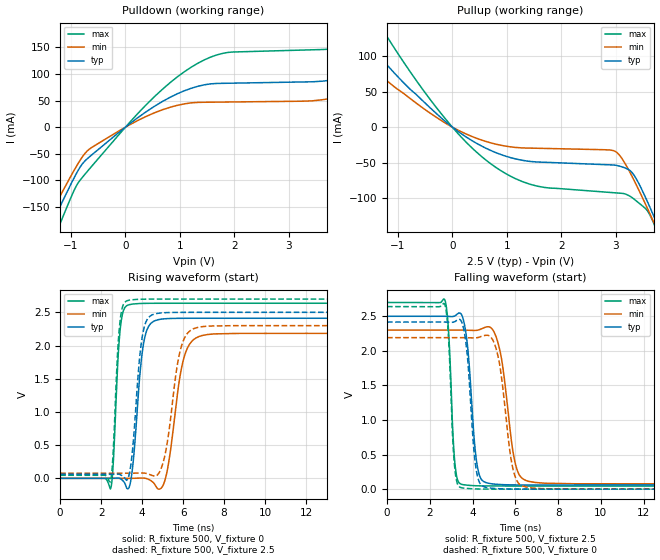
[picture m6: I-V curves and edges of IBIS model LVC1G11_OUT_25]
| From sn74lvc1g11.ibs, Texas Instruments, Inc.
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[Model]   LVC1G11_OUT_25
Model_type  Output
Vref =   0
Rref =   500
Cref =   30p
Vmeas =   1.25
| variable   typ   min   max
C_comp   8.68pF   6.47pF   11.64pF
| C_pullup   8.47pF   6.47pF   9.44pF
| C_pulldown   8.88pF   6.52pF   11.64pF
[Temperature Range]   40   100   -40
| Ambient temperature   25   85   -40
[Voltage range]   2.5   2.3   2.7
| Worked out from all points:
|   slope of the pulldown table from 0 to 0.375 V, typ, clamps not added: 13.1 ohm
|   slope of the pullup table from 0 to 0.375 V, typ, clamps not added: 19.1 ohm
|   rising waveform, R_fixture 500, V_fixture 0: 20-80 % time 389ps typ, 592ps min, 250ps max; typ from 0 V to 2.41 V
|   falling waveform, R_fixture 500, V_fixture 2.5: 20-80 % time 346ps typ, 532ps min, 224ps max; typ from 2.5 V to 0.06 V
|   rising waveform, R_fixture 500, V_fixture 2.5: 20-80 % time 383ps typ, 591ps min, 246ps max; typ from 0.06 V to 2.5 V
|   falling waveform, R_fixture 500, V_fixture 0: 20-80 % time 334ps typ, 507ps min, 221ps max; typ from 2.42 V to 0 V
[Pulldown]
| LVC1G11_OUT_25
|   Voltage   I(typ)   I(min)   I(max)
-5.5V     -1.065A    -962.2mA   -1.233A
-1.515V   -217.8mA   -190.9mA   -261.5mA
-1.145V   -137.3mA   -118.9mA   -167.6mA
-660mV    -55.79mA   -41.12mA   -78.48mA
535mV     39.4mA     27.09mA    57.66mA
1.455V    79.8mA     46.83mA    127mA
3.83V     89.86mA    55.41mA    148.1mA
5.34V     157.5mA    105.9mA    231.7mA
5.91V     188.7mA    52.63mA    283.1mA
6.525V    93.57mA    53.14mA    299.2mA
7.56V     94.12mA    54.12mA    161mA
11V       99.65mA    57.57mA    169.2mA
[Pullup]
| LVC1G11_OUT_25
|   Voltage   I(typ)   I(min)   I(max)
-5.5V     548.1mA    433.4mA    764.5mA
-2.31V    190.8mA    146mA      272.9mA
-1.86V    147mA      111.5mA    211.6mA
-1.295V   95.71mA    71.6mA     139.1mA
-180mV    11.41mA    8.219mA    16.71mA
710mV     -33.04mA   -22.25mA   -51.89mA
1.555V    -49.16mA   -29.78mA   -83.08mA
2.995V    -53.63mA   -34.3mA    -92.61mA
3.34V     -67.98mA   -75.27mA   -101.5mA
3.565V    -101.9mA   -111.4mA   -116.1mA
3.76V     -136.1mA   -144.4mA   -146.6mA
11V       -1.614A    -1.516A    -1.796A
[Ramp]
| LVC1G11_OUT_25
| variable   typ   min   max
dV/dt_r   1.54/4.17E-10   1.41/6.31E-10   1.68/2.67E-10
dV/dt_f   1.49/3.62E-10   1.36/5.51E-10   1.62/2.36E-10
R_load = 500
[Rising Waveform]
| LVC1G11_OUT_25
R_fixture =   500
C_fixture =   0
L_fixture =   0
V_fixture =   0
V_fixture_min = 0
V_fixture_max = 0
|   Time   V(typ)   V(min)   V(max)
0s        123.5pV    5.747nV    2.547nV
2.465ns   -41.49uV   4.441uV    -154.4mV
2.93ns    -4.546mV   -61.89uV   2.24V
3.375ns   -128.9mV   -44.43uV   2.615V
4.07ns    2.026V     3.747mV    2.635V
4.735ns   2.385V     -148.7mV   2.637V
5.21ns    2.405V     90.18mV    2.637V
6.065ns   2.41V      1.84V      2.637V
6.935ns   2.411V     2.151V     2.637V
34.99ns   2.411V     2.183V     2.637V
[Falling Waveform]
| LVC1G11_OUT_25
R_fixture =   500
C_fixture =   0
L_fixture =   0
V_fixture =   2.5
V_fixture_min = 2.3
V_fixture_max = 2.7
|   Time   V(typ)   V(min)   V(max)
0s        2.5V       2.3V       2.7V
2.705ns   2.5V       2.3V       2.737V
3.165ns   2.505V     2.3V       400.6mV
3.48ns    2.526V     2.3V       69.96mV
4.2ns     371mV      2.297V     49.1mV
4.695ns   88.9mV     2.349V     46.64mV
5.305ns   66.92mV    1.963V     45.91mV
6.02ns    61.5mV     342.5mV    45.73mV
6.63ns    60.51mV    112.6mV    45.69mV
34.99ns   60.09mV    77.08mV    45.62mV
[Rising Waveform]
| LVC1G11_OUT_25
R_fixture =   500
C_fixture =   0
L_fixture =   0
V_fixture =   2.5
V_fixture_min = 2.3
V_fixture_max = 2.7
|   Time   V(typ)   V(min)   V(max)
0s        60.06mV    77.04mV    45.59mV
2.45ns    60.01mV    77.04mV    -55.24mV
2.895ns   59.87mV    76.99mV    2.282V
3.34ns    23.31mV    77mV       2.681V
4ns       2.118V     80.7mV     2.698V
4.62ns    2.476V     32.88mV    2.7V
5.14ns    2.495V     384mV      2.7V
5.91ns    2.499V     1.981V     2.7V
6.7ns     2.5V       2.272V     2.7V
34.99ns   2.5V       2.3V       2.7V
[Falling Waveform]
| LVC1G11_OUT_25
R_fixture =   500
C_fixture =   0
L_fixture =   0
V_fixture =   0
V_fixture_min = 0
V_fixture_max = 0
|   Time   V(typ)   V(min)   V(max)
0s        2.416V     2.191V     2.64V
2.705ns   2.416V     2.191V     2.668V
3.16ns    2.421V     2.192V     326.1mV
3.495ns   2.414V     2.191V     18.92mV
4.155ns   314.3mV    2.189V     3.513mV
4.61ns    27.39mV    2.225V     1.138mV
5.22ns    6.589mV    1.878V     332.3uV
5.92ns    1.414mV    251.6mV    131.8uV
6.49ns    469.6uV    31.07mV    92.46uV
34.99ns   27.74uV    36.16uV    20.63uV
